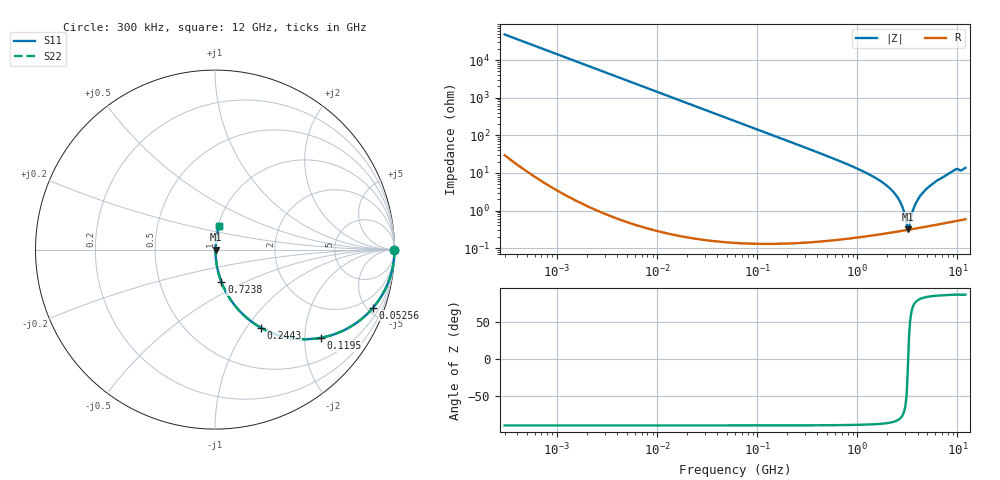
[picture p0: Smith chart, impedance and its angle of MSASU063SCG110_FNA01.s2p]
! MSASU063SCG110_FNA01  S-PARAMETER MODEL  ( Standard Model )
! Model Generated by TAIYO YUDEN Corporation (http://www.ty-top.com)
! Version 1.0
! TAIYO YUDEN Control No. 240819
! Copyright(c) 2024 TAIYO YUDEN CO.,LTD. All Rights Reserved.
! Product Description (link to TY-COMPAS)
! https://ds.yuden.co.jp/TYCOMPAS/or/detail?pn=MSASU063SCG110JFNA01&u=M
! Products Name : Multilayer Ceramic Capacitors
! Characteristics :
!  Capacitance : 11 [pF] , Rated Voltage : 50 [V] , TCC : CG / C0G
!  Case Size : 0.6 x 0.3 / 0.024 x 0.012 [mm/inch] , Thickness : 0.3 / 0.012 [mm/inch]
!  (Conditions: Temperature = 25 [degC] , DC Bias Voltage = 0 [V])
! External Node Assignments :
!  1  o---| |---o  2
! GND o---------o GND
! Frequency Range : 0.3MHz  -  12000MHz  [ 401 STEP ]
# MHZ S RI R 50
! Freq[MHz].  S11 Real  S11 Imag  S21 Real  S21 Imag  S12 Real  S12 Imag  S22 Real  S22 Imag
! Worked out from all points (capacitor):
!   401 points, 300 kHz to 12 GHz, reference 50 ohm
!   read as one part in series: C = 11.1 pF near 316.3 kHz
!   lowest |Z| = 316 mohm at 3.191 GHz (marker M1)
!   series resonance near 3.218 GHz, so ESL is about 220 pH
!   S11 on the Smith chart (normalised r, x): 300 kHz: open; 52.56 MHz: 1.00, -5.46; 119.5 MHz: 1.00, -2.40; 244.3 MHz: 1.00, -1.17; 723.8 MHz: 1.00, -0.38; 12 GHz: 1.01, +0.27
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0.3  1 -0.00209  5.65e-06 0.00209  5.65e-06 0.00209  1 -0.00209
1.769972  0.9998 -0.0123  0.000154 0.0123  0.000154 0.0123  0.9998 -0.0123
10.44266  0.9947 -0.0723  0.00527 0.0723  0.00527 0.0723  0.9947 -0.0723
24.37677  0.9719 -0.165  0.0281 0.165  0.0281 0.165  0.9719 -0.165
52.55639  0.8817 -0.3227  0.1183 0.3227  0.1183 0.3227  0.8817 -0.3227
60  0.8512 -0.3556  0.1488 0.3556  0.1488 0.3556  0.8512 -0.3556
119.4772  0.5902 -0.4913  0.4098 0.4913  0.4098 0.4913  0.5902 -0.4913
244.3004  0.2551 -0.4348  0.7449 0.4348  0.7449 0.4348  0.2551 -0.4348
353.9943  0.1393 -0.3445  0.8607 0.3445  0.8607 0.3445  0.1393 -0.3445
723.8279  0.0358 -0.1814  0.9642 0.1814  0.9642 0.1814  0.0358 -0.1814
1403.667  0.00895 -0.0821  0.991 0.0821  0.991 0.0821  0.00895 -0.0821
2088.533  0.00412 -0.0397  0.9959 0.0397  0.9959 0.0397  0.00412 -0.0397
2650.866  0.00312 -0.0176  0.9969 0.0176  0.9969 0.0176  0.00312 -0.0176
2870.14  0.00302 -0.0104  0.997 0.0104  0.997 0.0104  0.00302 -0.0104
3107.553  0.00303 -0.0034  0.997 0.0034  0.997 0.0034  0.00303 -0.0034
3190.978  0.00305 -0.000781  0.9969 0.000781  0.9969 0.000781  0.00305 -0.000781
3364.605  0.00314 0.0039  0.9969 -0.0039  0.9969 -0.0039  0.00314 0.0039
3642.919  0.00336 0.0108  0.9966 -0.0108  0.9966 -0.0108  0.00336 0.0108
3944.255  0.00367 0.0175  0.9963 -0.0175  0.9963 -0.0175  0.00367 0.0175
4875.354  0.00507 0.0367  0.9949 -0.0367  0.9949 -0.0367  0.00507 0.0367
9207.246  0.0183 0.1137  0.9817 -0.1137  0.9817 -0.1137  0.0183 0.1137
12000  0.0237 0.1323  0.9763 -0.1323  0.9763 -0.1323  0.0237 0.1323
